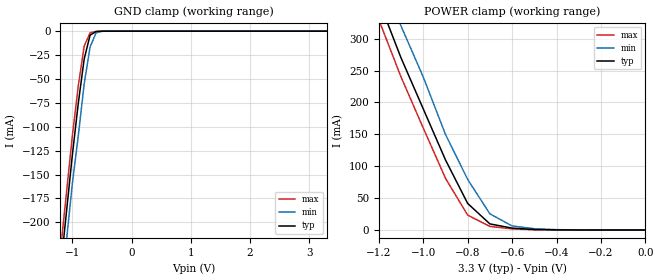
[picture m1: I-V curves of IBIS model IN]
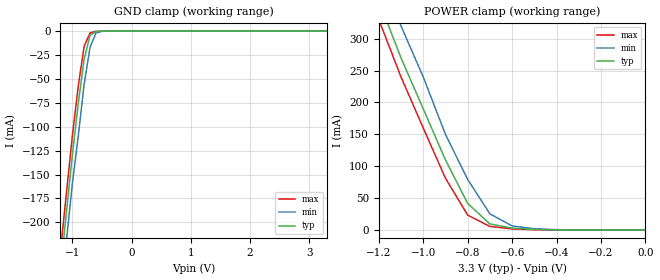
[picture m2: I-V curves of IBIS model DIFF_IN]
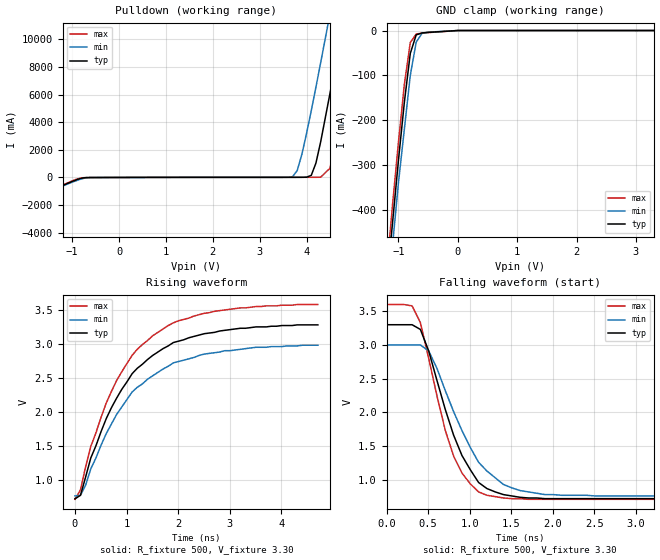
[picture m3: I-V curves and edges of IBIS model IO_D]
| Integrated Devices Technolgy, Inc
[Ibis Ver]   4.2
[File Name]   9zxl1550d.ibs
[Source]   Integrated Devices Technolgy, Inc.
[Notes]   Rev 1.0 created by EvK
[File Rev]   1.0
[Date]   Thursday, Mar 22, 2018
[Disclaimer] Integrated Device Technology, Inc. ("IDT") hereby grants the
   user of this IBIS model a non-exclusive, nontransferable
   license to use this IBIS model under the following terms. The
   user is granted this license only to use the IBIS model and is
   not granted rights to sell, copy (except as needed to run the
   IBIS model), rent, lease or sub-license the IBIS model in
   whole or in part, or in modified form to anyone. The User may
   modify the IBIS model to suit its specific applications, but
   rights to derivative works and such modifications shall belong
   to IDT. This IBIS model is provided on an AS IS" basis and IDT
   makes absolutely no warranty with respect to the information
   contained herein. IDT DISCLAIMS AND CUSTOMER WAIVES ALL
   WARRANTIES, EXPRESS AND IMPLIED, INCLUDING WARRANTIES OF
   MERCHANTABILITY AND FITNESS FOR A PARTICULAR PURPOSE. THE
   ENTIRE RISK AS TO QUALITY AND PERFORMANCE IS WITH THE USER
   ACCORDINGLY, IN NO EVENT SHALL IDT BE LIABLE FOR ANY DIRECT OR
   INDIRECT DAMAGES, WHETHER IN CONTRACT OR TORT, INCLUDING ANY
   LOST PROFITS OR OTHER INCIDENTAL, CONSEQUENTIAL, EXEMPLARY, OR
   PUNITIVE DAMAGES ARISING OUT OF THE USE OR APPLICATION OF THE
   IBIS model. Further, IDT reserves the right to make changes
   without notice to any product herein to improve reliability,
   function, or design. IDT does not convey any license under
   patent rights or any other intellectual property rights,
   including those of third parties. IDT is not obligated to
   provide maintenance or support for the licensed IBIS model.
[Disclaimer]   (C) Copyright Integrated Device Technology, Inc. 2010 All
   rights reserved
|   COMPONENT: 9ZXL1550D
[Component]   9ZXL1550
[Manufacturer]   Integrated Device Technology, Inc.
[Package]
| variable   typ   min   max
R_pkg   81.10m   62.20m   100.00m
L_pkg   6.70nH   4.90nH   8.50nH
C_pkg   0.53pF   0.21pF   0.85pF
[Pin]   signal_name   model_name   R_pin   L_pin   C_pin
1   VDDA   POWER
2   GNDA   GND
3   100M_133M#   IN
4   HIBW_BYPM_LOBW#   IN
5   CKPWRGD_PD#   IN
6   GND   GND
7   VDDR   POWER
8   DIF_IN   DIFF_IN
9   DIF_IN#   DIFF_IN
10   SADR0_tri   IN
11   SMBDAT   IO_D
12   SMBCLK   IN_D
13   SADR1_tri   IN
14   FBOUT_NC#   LP_HCSL85
15   FBOUT_NC   LP_HCSL85
16   GND   GND
17   DIF_0   LP_HCSL85
18   DIF_0#   LP_HCSL85
19   VDDIO   POWER
20   GND   GND
21   DIF_1   LP_HCSL85
22   DIF_1#   LP_HCSL85
23   DIF_2   LP_HCSL85
24   DIF_2#   LP_HCSL85
25   GND   GND
26   VDD   POWER
27   DIF_3   LP_HCSL85
28   DIF_3#   LP_HCSL85
29   DIF_4   LP_HCSL85
30   DIF_4#   LP_HCSL85
31   VDDIO   POWER
32   GND   GND
33   DIF_5   LP_HCSL85
34   DIF_5#   LP_HCSL85
35   GND   GND
36   VDDIO   POWER
37   DIF_6   LP_HCSL85
38   DIF_6#   LP_HCSL85
39   DIF_7   LP_HCSL85
40   DIF_7#   LP_HCSL85
41   VDD   POWER
42   GND   GND
43   DIF_8   LP_HCSL85
44   DIF_8#   LP_HCSL85
45   DIF_9   LP_HCSL85
46   DIF_9#   LP_HCSL85
47   GND   GND
48   VDDIO   POWER
49   DIF_10   LP_HCSL85
50   DIF_10#   LP_HCSL85
51   VDDIO   POWER
52   GND   GND
53   DIF_11   LP_HCSL85
54   DIF_11#   LP_HCSL85
55   DIF_12   LP_HCSL85
56   DIF_12#   LP_HCSL85
57   GND   GND
58   VDD   POWER
59   DIF_13   LP_HCSL85
60   DIF_13#   LP_HCSL85
61   DIF_14   LP_HCSL85
62   DIF_14#   LP_HCSL85
63   VDDIO   POWER
64   GND   GND
65   EPAD   GND
[Diff Pin]   inv_pin   vdiff   tdelay_typ
8   9   NA   NA
15   14   NA   NA
17   18   NA   NA
21   22   NA   NA
23   24   NA   NA
27   28   NA   NA
29   30   NA   NA
33   34   NA   NA
37   38   NA   NA
39   40   NA   NA
43   44   NA   NA
45   46   NA   NA
49   50   NA   NA
53   54   NA   NA
55   56   NA   NA
59   60   NA   NA
61   62   NA   NA
| Models and submodels in the file (5): IN (Input), DIFF_IN (Input), IO_D (I/O_open_drain), IN_D (Input), LP_HCSL85 (Output)
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|   Model IN
[Model]   IN
Model_type   Input
Polarity   Inverting
Enable   Active-High
Vinl =   1.00V
Vinh =   2.00V
C_comp   3.40pF   2.85pF   3.95pF
[Temperature Range]   27.00   70.00   0.000
[Voltage Range]   3.30V   3.00V   3.60V
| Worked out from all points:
|   GND clamp passes 1 mA (typ) near -0.62 V on its own axis
|   POWER clamp passes 1 mA (typ) near -0.51 V on its own axis
[GND_clamp]
| voltage   I(typ)   I(min)   I(max)
-3.3V     -1.54A     -1.54A     -1.54A
-1.2V     -250mA     -270mA     -230mA
-1.1V     -190mA     -220mA     -170mA
-1V       -130mA     -160mA     -110mA
-900mV    -75.97mA   -110mA     -57.72mA
-800mV    -29.3mA    -55.39mA   -15.7mA
-700mV    -4.2mA     -16.67mA   -1.77mA
-600mV    -420uA     -1.81mA    -210uA
-500mV    -36.28uA   -150uA     -14.74uA
3.3V      150pA      92.22uA    -1.21nA
[POWER_clamp]
| voltage   I(typ)   I(min)   I(max)
-3.3V     2.31A      2.35A      2.29A
-1.2V     360mA      410mA      330mA
-1.1V     270mA      320mA      240mA
-1V       190mA      240mA      160mA
-900mV    110mA      150mA      81.19mA
-800mV    41.59mA    79.25mA    23.27mA
-700mV    9.51mA     25.32mA    5.62mA
-600mV    2.91mA     6.31mA     1.67mA
-500mV    750uA      1.96mA     350uA
-300mV    20.87uA    92.22uA    6.56uA
0V        150pA      200pA      160pA
|   Model DIFF_IN
[Model]   DIFF_IN
Model_type   Input
Polarity   Inverting
Enable   Active-High
Vinl =   0.200V
Vinh =   0.500V
|   Input threshold is differential cross-over voltage
C_comp   3.40pF   2.85pF   3.95pF
[Temperature Range]   27.00   70.00   0.000
[Voltage Range]   3.30V   3.00V   3.60V
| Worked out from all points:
|   GND clamp passes 1 mA (typ) near -0.62 V on its own axis
|   POWER clamp passes 1 mA (typ) near -0.51 V on its own axis
[GND_clamp]
| voltage   I(typ)   I(min)   I(max)
-3.3V     -1.54A     -1.54A     -1.54A
-1.2V     -250mA     -270mA     -230mA
-1.1V     -190mA     -220mA     -170mA
-1V       -130mA     -160mA     -110mA
-900mV    -75.97mA   -110mA     -57.72mA
-800mV    -29.3mA    -55.39mA   -15.7mA
-700mV    -4.2mA     -16.67mA   -1.77mA
-600mV    -420uA     -1.81mA    -210uA
-500mV    -36.28uA   -150uA     -14.74uA
3.3V      150pA      92.22uA    -1.21nA
[POWER_clamp]
| voltage   I(typ)   I(min)   I(max)
-3.3V     2.31A      2.35A      2.29A
-1.2V     360mA      410mA      330mA
-1.1V     270mA      320mA      240mA
-1V       190mA      240mA      160mA
-900mV    110mA      150mA      81.19mA
-800mV    41.59mA    79.25mA    23.27mA
-700mV    9.51mA     25.32mA    5.62mA
-600mV    2.91mA     6.31mA     1.67mA
-500mV    750uA      1.96mA     350uA
-300mV    20.87uA    92.22uA    6.56uA
0V        150pA      200pA      160pA
|   Model IO_D
[Model]   IO_D
Model_type   I/O_open_drain
Polarity   Non-Inverting
Enable   Active-High
Vinl =   1.00V
Vinh =   2.00V
Vmeas =   1.650V
Cref =   2.00pF
Rref =  500.000
Vref =   1.660V
C_comp   3.40pF   2.85pF   3.95pF
[Temperature Range]   27.00   70.00   0.000
[Voltage Range]   3.30V   3.00V   3.60V
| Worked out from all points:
|   slope of the pulldown table from 0 to 0.495 V, typ, clamps not added: 131 ohm
|   GND clamp passes 1 mA (typ) near -0.12 V on its own axis
|   rising waveform, R_fixture 500, V_fixture 3.30: 20-80 % time 1.13ns typ, 1.18ns min, 1.1ns max; typ from 0.72 V to 3.28 V
|   falling waveform, R_fixture 500, V_fixture 3.30: 20-80 % time 430ps typ, 510ps min, 367ps max; typ from 3.3 V to 0.72 V
[Pulldown]
| voltage   I(typ)   I(min)   I(max)
-3.3V     -3.78A     -3.65A     -3.87A
-800mV    -50.99mA   -100mA     -26.91mA
3.7V      9.44mA     53.55mA    11.23mA
3.8V      10.07mA    490mA      11.25mA
3.9V      12.32mA    1.67A      11.27mA
4.1V      150mA      4.83A      11.65mA
4.3V      2.56A      8.29A      17.33mA
4.5V      6.09A      11.85A     670mA
4.7V      9.81A      15.47A     3.91A
4.9V      13.62A     19.11A     7.69A
5.1V      17.46A     22.78A     11.6A
6.6V      46.76A     50.55A     41.81A
[GND_clamp]
| voltage   I(typ)   I(min)   I(max)
-3.3V     -3.78A     -3.65A     -3.87A
-1.2V     -570mA     -610mA     -540mA
-1.1V     -430mA     -480mA     -390mA
-1V       -290mA     -340mA     -250mA
-900mV    -160mA     -220mA     -120mA
-800mV    -50.99mA   -100mA     -26.91mA
-700mV    -9.68mA    -25.77mA   -7.84mA
-600mV    -5.33mA    -5.93mA    -5.63mA
0V        0A         0A         0A
3.3V      150pA      220pA      150pA
[Ramp]
| variable   typ   min   max
dV/dt_r   1.54/1.11n   1.33/1.16n   1.72/1.07n
dV/dt_f   1.55/0.42n   1.34/0.53n   1.73/0.36n
R_load = 500
[Rising Waveform]
R_fixture = 500
V_fixture = 3.30
V_fixture_min = 3.00
V_fixture_max = 3.60
| time   V(typ)   V(min)   V(max)
|  0.000S   0.72V   0.76V   0.71V
|1.000e-10S   0.72V   0.76V   0.71V
|   0.20nS   0.72V   0.76V   0.71V
|   0.30nS   0.72V   0.76V   0.72V
|   0.40nS   0.77V   0.77V   0.85V
|   0.50nS   1.04V   0.92V   1.19V
|   0.60nS   1.32V   1.16V   1.49V
|   0.70nS   1.50V   1.32V   1.69V
|   0.80nS   1.71V   1.51V   1.92V
|   0.90nS   1.90V   1.68V   2.13V
|   1.00nS   2.06V   1.82V   2.30V
|   1.10nS   2.20V   1.96V   2.46V
|   1.20nS   2.33V   2.07V   2.59V
|   1.30nS   2.44V   2.18V   2.71V
|   1.40nS   2.56V   2.29V   2.83V
|   1.50nS   2.64V   2.36V   2.92V
|   1.60nS   2.70V   2.41V   2.99V
|   1.70nS   2.77V   2.48V   3.05V
|   1.80nS   2.83V   2.53V   3.12V
|   1.90nS   2.88V   2.58V   3.17V
|   2.00nS   2.93V   2.63V   3.22V
|   2.10nS   2.97V   2.67V   3.27V
|   2.20nS   3.02V   2.72V   3.31V
|   2.30nS   3.04V   2.74V   3.34V
|   2.40nS   3.06V   2.76V   3.36V
|   2.50nS   3.09V   2.78V   3.38V
|   2.60nS   3.11V   2.80V   3.41V
|   2.70nS   3.13V   2.83V   3.43V
|   2.80nS   3.15V   2.85V   3.45V
|   2.90nS   3.16V   2.86V   3.46V
|   3.00nS   3.17V   2.87V   3.48V
|   3.10nS   3.19V   2.88V   3.49V
|   3.20nS   3.20V   2.90V   3.50V
|   3.30nS   3.21V   2.90V   3.51V
|   3.40nS   3.22V   2.91V   3.52V
|   3.50nS   3.23V   2.92V   3.53V
|   3.60nS   3.23V   2.93V   3.53V
|   3.70nS   3.24V   2.94V   3.54V
|   3.80nS   3.25V   2.95V   3.55V
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0s        720mV      760mV      710mV
107.7ps   770mV      770mV      850mV
307.7ps   1.32V      1.16V      1.49V
607.7ps   1.9V       1.68V      2.13V
807.7ps   2.2V       1.96V      2.46V
1.108ns   2.56V      2.29V      2.83V
1.508ns   2.83V      2.53V      3.12V
1.908ns   3.02V      2.72V      3.31V
2.708ns   3.17V      2.87V      3.48V
4.708ns   3.28V      2.98V      3.58V
[Falling Waveform]
R_fixture = 500
V_fixture = 3.30
V_fixture_min = 3.00
V_fixture_max = 3.60
| time   V(typ)   V(min)   V(max)
|  0.000S   3.30V   3.00V   3.60V
|1.000e-10S   3.30V   3.00V   3.60V
|   0.20nS   3.30V   3.00V   3.60V
|   0.30nS   3.30V   3.00V   3.60V
|   0.40nS   3.30V   3.00V   3.60V
|   0.50nS   3.30V   3.00V   3.60V
|   0.60nS   3.30V   3.00V   3.58V
|   0.70nS   3.23V   3.00V   3.33V
|   0.80nS   2.91V   2.91V   2.80V
|   0.90nS   2.47V   2.65V   2.24V
|   1.00nS   2.04V   2.32V   1.73V
|   1.10nS   1.66V   2.01V   1.35V
|   1.20nS   1.36V   1.73V   1.10V
|   1.30nS   1.15V   1.48V   0.94V
|   1.40nS   0.96V   1.26V   0.82V
|   1.50nS   0.87V   1.13V   0.77V
|   1.60nS   0.82V   1.03V   0.75V
|   1.70nS   0.78V   0.93V   0.73V
|   1.80nS   0.76V   0.88V   0.72V
|   1.90nS   0.74V   0.84V   0.72V
|   2.00nS   0.73V   0.82V   0.71V
|   2.10nS   0.73V   0.80V   0.71V
|   2.20nS   0.72V   0.78V   0.71V
|   2.30nS   0.72V   0.78V   0.71V
|   2.40nS   0.72V   0.77V   0.71V
|   2.50nS   0.72V   0.77V   0.71V
|   2.60nS   0.72V   0.77V   0.71V
|   2.70nS   0.72V   0.77V   0.71V
|   2.80nS   0.72V   0.76V   0.71V
|   2.90nS   0.72V   0.76V   0.71V
|   3.00nS   0.72V   0.76V   0.71V
|   3.10nS   0.72V   0.76V   0.71V
|   3.20nS   0.72V   0.76V   0.71V
|   3.30nS   0.72V   0.76V   0.71V
|   3.40nS   0.72V   0.76V   0.71V
|   3.50nS   0.72V   0.76V   0.71V
|   3.60nS   0.72V   0.76V   0.71V
|   3.70nS   0.72V   0.76V   0.71V
|   3.80nS   0.72V   0.76V   0.71V
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0s        3.3V       3V         3.6V
307.7ps   3.3V       3V         3.58V
407.7ps   3.23V      3V         3.33V
507.7ps   2.91V      2.91V      2.8V
707.7ps   2.04V      2.32V      1.73V
807.7ps   1.66V      2.01V      1.35V
1.108ns   960mV      1.26V      820mV
1.408ns   780mV      930mV      730mV
1.908ns   720mV      780mV      710mV
4.708ns   720mV      760mV      710mV
